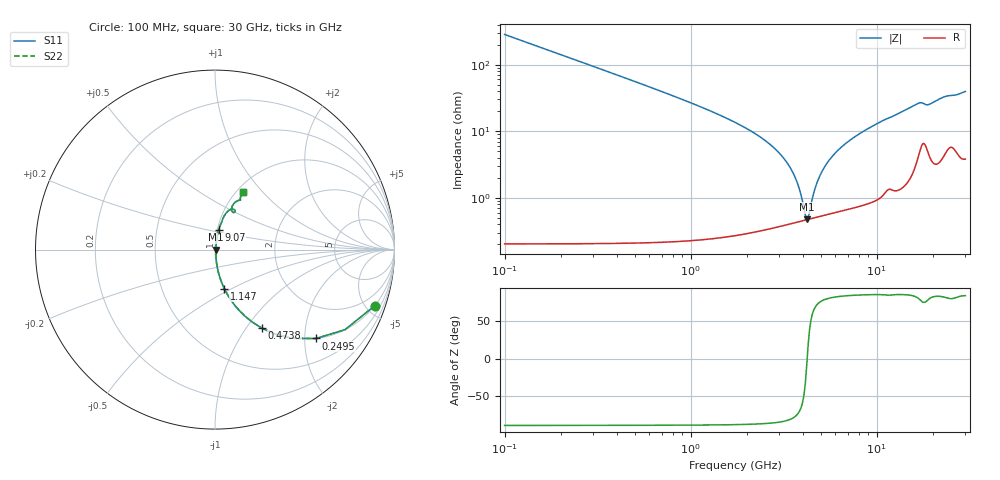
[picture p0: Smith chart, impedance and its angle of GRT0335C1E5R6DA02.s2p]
!Murata Part Number: GRT0335C1E5R6DA02
!These Parameters are Measured in Series Mode Connection
!Data Generated on Jun 19, 2026
!  o--ll--o
!Port1  Port2
!  o------o
!Operation Temp=25[degC], DC Bias Voltage=0[V]
!Freq. Start=100[MHz] Stop=30[GHz] 401[Steps]
# Hz S RI R 50
!Freq.(Hz) S11(Real) S11(Imag) S21(Real) S21(Imag) S12(Real) S12(Imag) S22(Real) S22(Imag)
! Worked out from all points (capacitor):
!   401 points, 100 MHz to 30 GHz, reference 50 ohm
!   read as one part in series: C = 5.6 pF near 249.5 MHz
!   lowest |Z| = 474 mohm at 4.211 GHz (marker M1)
!   series resonance near 4.233 GHz, so ESL is about 250 pH
!   S11 on the Smith chart (normalised r, x): 100 MHz: 1.00, -5.68; 249.5 MHz: 1.00, -2.27; 473.8 MHz: 1.00, -1.18; 1.147 GHz: 1.00, -0.46; 9.07 GHz: 1.02, +0.22; 30 GHz: 1.08, +0.79
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1e8  0.8895 -0.3131  0.1105 0.3131  0.1105 0.3131  0.8895 -0.3131
2.495e8  0.5629 -0.4951  0.4371 0.4951  0.4371 0.4951  0.5629 -0.4951
4.7375e8  0.2604 -0.4371  0.7396 0.4371  0.7396 0.4371  0.2604 -0.4371
7.7275e8  0.1135 -0.3142  0.8865 0.3142  0.8865 0.3142  0.1135 -0.3142
1.1465e9  0.0519 -0.2168  0.9481 0.2168  0.9481 0.2168  0.0519 -0.2168
1.96875e9  0.0153 -0.1105  0.9847 0.1105  0.9847 0.1105  0.0153 -0.1105
3.2395e9  0.00516 -0.0356  0.9948 0.0356  0.9948 0.0356  0.00516 -0.0356
3.688e9  0.00458 -0.0182  0.9954 0.0182  0.9954 0.0182  0.00458 -0.0182
4.06175e9  0.00458 -0.00542  0.9954 0.00542  0.9954 0.00542  0.00458 -0.00542
4.21125e9  0.00467 -0.000676  0.9953 0.000676  0.9953 0.000676  0.00467 -0.000676
4.36075e9  0.0048 0.00389  0.9952 -0.00389  0.9952 -0.00389  0.0048 0.00389
4.7345e9  0.00529 0.0147  0.9947 -0.0147  0.9947 -0.0147  0.00529 0.0147
5.10825e9  0.00596 0.0247  0.994 -0.0247  0.994 -0.0247  0.00596 0.0247
5.70625e9  0.00734 0.0394  0.9927 -0.0394  0.9927 -0.0394  0.00734 0.0394
6.5285e9  0.00972 0.0579  0.9903 -0.0579  0.9903 -0.0579  0.00972 0.0579
9.07e9  0.02 0.1077  0.98 -0.1077  0.98 -0.1077  0.02 0.1077
1.01165e10  0.0257 0.1265  0.9743 -0.1265  0.9743 -0.1265  0.0257 0.1265
1.505e10  0.064 0.2061  0.936 -0.2061  0.936 -0.2061  0.064 0.2061
1.75915e10  0.112 0.2159  0.888 -0.2159  0.888 -0.2159  0.112 0.2159
2.005825e10  0.0935 0.2349  0.9065 -0.2349  0.9065 -0.2349  0.0935 0.2349
2.50665e10  0.1424 0.2749  0.8576 -0.2749  0.8576 -0.2749  0.1424 0.2749
3e10  0.1581 0.3197  0.8419 -0.3197  0.8419 -0.3197  0.1581 0.3197
